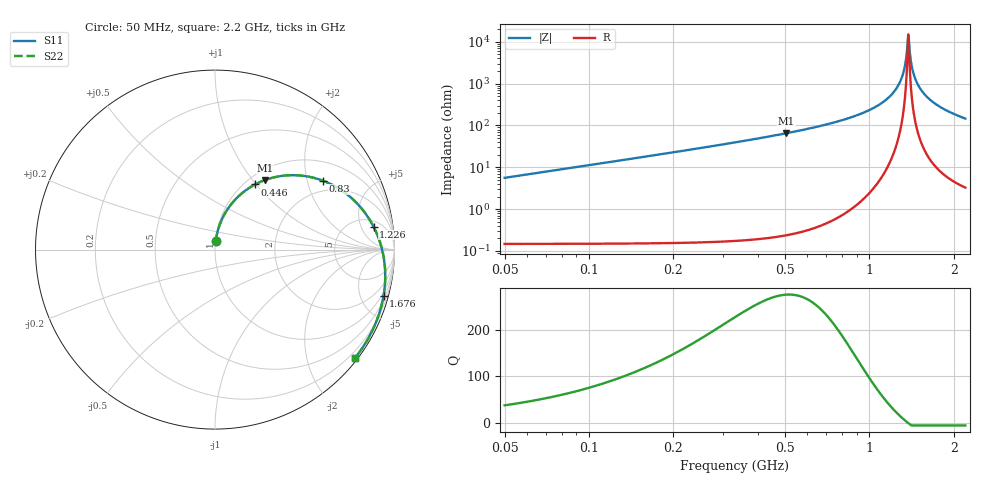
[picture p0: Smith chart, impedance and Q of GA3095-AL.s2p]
! Coilcraft GA3095-AL Air Core Inductor
! 01 July 2008
# MHZ S MA R 50
!Freq  MagS11  AngS11  MagS21  AngS21  MagS12  AngS12  MagS22  AngS22
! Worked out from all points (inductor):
!   360 points, 50 MHz to 2.2 GHz, reference 50 ohm
!   read as 1/Y11, port 2 shorted: L = 17.8 nH near 56 MHz
!   highest Q = 275 at 506 MHz (marker M1), where L = 20.5 nH
!   self-resonance near 1.376 GHz
!   S11 on the Smith chart (normalised r, x): 50 MHz: 1.00, +0.10; 446 MHz: 1.11, +0.99; 830 MHz: 1.61, +2.51; 1.226 GHz: 7, +9; 1.676 GHz: 0.76, -7.40; 2.2 GHz: 0.06, -2.92
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50  0.04987 84.8  0.9973 -3.5  0.9973 -3.5  0.04991 84.8
74  0.07375 83.6  0.9958 -5.2  0.9958 -5.2  0.0738 83.6
98  0.09757 82.2  0.9938 -6.9  0.9938 -6.9  0.09764 82.2
170  0.1685 77.5  0.9842 -12.0  0.9842 -12.0  0.1687 77.5
272  0.2671 70.5  0.9622 -19.2  0.9622 -19.2  0.2673 70.5
410  0.3946 60.9  0.9173 -28.9  0.9173 -28.9  0.3948 60.9
446  0.4264 58.4  0.9029 -31.4  0.9029 -31.4  0.4267 58.4
506  0.4778 54.2  0.8767 -35.6  0.8767 -35.6  0.4781 54.2
638  0.583 45.2  0.8102 -44.6  0.8102 -44.6  0.5834 45.2
770  0.676 36.4  0.734 -53.3  0.734 -53.3  0.6764 36.4
830  0.7138 32.5  0.6969 -57.2  0.6969 -57.2  0.7143 32.5
1130  0.86 13.8  0.5018 -75.7  0.5018 -75.7  0.8606 13.8
1226  0.8924 8.2  0.4398 -81.1  0.4398 -81.1  0.893 8.2
1484  0.951 -5.8  0.2846 -94.3  0.2846 -94.3  0.9516 -5.8
1676  0.9735 -15.2  0.1849 -102.5  0.1849 -102.5  0.9741 -15.2
1844  0.9832 -22.9  0.1108 -107.6  0.1108 -107.6  0.9838 -22.9
1940  0.9858 -27.1  0.07433 -108.6  0.07433 -108.6  0.9864 -27.1
2018  0.9868 -30.4  0.04805 -106.4  0.04805 -106.4  0.9873 -30.4
2078  0.987 -32.9  0.03029 -99.4  0.03029 -99.4  0.9876 -32.9
2162  0.9867 -36.3  0.01332 -54.0  0.01332 -54.0  0.9873 -36.3
2180  0.9866 -37.0  0.01283 -34.2  0.01283 -34.2  0.9872 -37.0
2200  0.9864 -37.8  0.01414 -14.2  0.01414 -14.2  0.987 -37.8
